FUNCTION_BLOCK FB_Visu
VAR_INPUT
	(***** Sensors to detect boxes *****)
	bBarrierSensor				AT %I*: BOOL;	// True if barrier sensor detects a box
	bMetalSensor				AT %I*: BOOL;	// True if metal sensor detects a metal box
	bPlasticSensor				AT %I*: BOOL;	// True if plastic sensor detects a box
	
	bError						: BOOL;			// True if modules have errors
(***** Axis variables *****)
	lrAxisVelo					: LREAL;
	
(***** State of machine elements *****)
	bComprAirEnabled			: BOOL;			// True if compressed air is enabled
	bPowerEnabled				: BOOL;			// True if power supply is enabled
	bMainAxisMoves				: BOOL;			// True if main axis is moving
	bMetalAxisMoves				: BOOL;			// True if metal axis is moving
	bPlasticAxisMoves			: BOOL;			// True if plastic axis is moving
	bClampToWork				: BOOL;			// True if clamp cylinder moves to work position
	bBarrierToWork				: BOOL;			// True if barrier cylinder moves to work position
	bMetalToWork				: BOOL;			// True if metal cylinder moves to work position
	bPlasticToWork				: BOOL;			// True if plastic cylinder moves to work position
(***** Error *****)
	bClampError					: BOOL;			// True if clamp cylinder has an error
	sClampErrMsg				: STRING;			// Error message of clamp cylinder
	bMetalCylError				: BOOL;			// True if metal cylinder has an error
	sMetalErrMsg				: STRING;			// Error message of metal cylinder
	bPlasticCylError			: BOOL;			// True if plastic cylinder has an error
	sPlasticErrMsg				: STRING;			// Error message of plastic cylinder
	iMainAxisErrorId			: DWORD;			// Error id of main axis
	iMetalAxisErrorId			: DWORD;			// Error id of metal axis
	iPlasticAxisErrorId			: DWORD;			// Error id of plastic axis
	
(***** PS_PackML_StateMachine *****)
	bStarted					: BOOL;			// True if state machine is in state EXECUTE
	bStopped					: BOOL;			// True if state machine is in state STOPPED
	bReset						: BOOL;			// True if state machine is in state RESETTING
	bAborted					: BOOL;			// True if state machine is in state ABORTED
	bIdle						: BOOL;			// True if state machine is in state IDLE
	bAuto						: BOOL;			// True if state machine is in mode AUTOMATIC
	bSemi						: BOOL;			// True if state machine is in mode SEMIAUTOMATIC
	bManual						: BOOL;			// True if state machine is in mode MANUAL
	bMaintenance				: BOOL;			// True if state machine is in mode MAINTENANCE
	bStartButtonOff				: BOOL;			// To turn off start button

(***** Buttons of visualisation - inputs *****)
		(* State buttons *)
	bButtonPowerIn				: BOOL;			// Input signal of power button
	bButtonComprAirIn			: BOOL;			// Input signal of compressed air button
	bButtonStartIn				: BOOL;			// Input signal of start button
	bButtonStopIn				: BOOL;			// Input signal of stop button
	bButtonResetIn				: BOOL;			// Input signal of reset button
	bButtonAbortIn				: BOOL;			// Input signal of abort button
		(* Mode buttons *)
	bButtonAutoIn				: BOOL;			// Input signal of automatic button
	bButtonSemiIn				: BOOL;			// Input signal of semi-automatic button
	bButtonManuIn				: BOOL;			// Input signal of manual button
	bButtonMaintenanceIn		: BOOL;			// Input signal of maintenance button
		(* Axis buttons *)
	bButtonMainFwIn				: BOOL;			// Input signal of button to move main axis forwards
	bButtonMainBwIn				: BOOL;			// Input signal of button to move main axis backwards
	bButtonMetalFwIn			: BOOL;			// Input signal of button to move metal axis forwards
	bButtonMetalBwIn			: BOOL;			// Input signal of button to move metal axis backwards
	bButtonPlasticFwIn			: BOOL;			// Input signal of button to move plastic axis forwards
	bButtonPlasticBwIn			: BOOL;			// Input signal of button to move plastic axis backwards
		(* Cylinder buttons *)
	bButtonClampToWorkIn		: BOOL;			// Input signal of button to move clamp cylinder
	bButtonBarrierToWorkIn		: BOOL;			// Input signal of button to move barrier cylinder
	bButtonMetalToWorkIn		: BOOL;			// Input signal of button to move metal cylinder
	bButtonPlasticToWorkIn		: BOOL;			// Input signal of button to move plastic cylinder
END_VAR
VAR_OUTPUT
	lrYClamp					AT %Q*: LREAL;					// Y-Coordinate of clamp cylinder
	lrYBarrier					AT %Q*: LREAL;					// Y-Coordinate of barrier cylinder
	lrYMetal					AT %Q*: LREAL;					// Y-Coordinate of metal cylinder
	lrYPlastic					AT %Q*: LREAL;					// Y-Coordinate of plastic cylinder
	lrBoxX						AT %Q*: ARRAY[1..4] OF LREAL;	// X-Coordinates of boxes
	lrBoxY						AT %Q*: ARRAY[1..4] OF LREAL;	// Y-Coordinates of boxes
	
(***** Buttons of visualisation - outputs *****)
		(* State buttons *)
	bButtonPowerOut				: BOOL;			// To turn on and off the machine
	bButtonComprAirOut			: BOOL;			// To enable compressed air
	bButtonStartOut				: BOOL;			// To change state into state START
	bButtonStopOut				: BOOL;			// To change state into state STOP
	bButtonResetOut				: BOOL;			// To change state into state RESET
	
		(* Mode buttons *)
	bButtonAutoOut				: BOOL;			// To change mode into mode AUTOMATIC		
	bButtonSemiOut				: BOOL;			// To change mode into mode SEMI-AUTOMATIC	
	bButtonManuOut				: BOOL;			// To change mode into mode MANAUL	
	bButtonMaintenanceOut		: BOOL;			// To change mode into mode MAINTENANCE	
	
		(* Axis buttons *)
	bButtonMainFwOut			: BOOL;			// To move main axis forwards
	bButtonMainBwOut			: BOOL;			// To move main axis backwards
	bButtonMetalFwOut			: BOOL;			// To move metal axis forwards
	bButtonMetalBwOut			: BOOL;			// To move metal axis backwards
	bButtonPlasticFwOut			: BOOL;			// To move plastic axis forwards
	bButtonPlasticBwOut			: BOOL;			// To move plastic axis backwards
	
		(* Cylinder buttons *)
	bButtonClampToWorkOut		: BOOL;			// To move manually clamp cylinder to work position
	bButtonBarrierToWorkOut		: BOOL;			// To move manually barrier cylinder to work position
	bButtonMetalToWorkOut		: BOOL;			// To move manually metal cylinder to work position
	bButtonPlasticToWorkOut		: BOOL;			// To move manually plastic cylinder to work position
END_VAR
VAR
	iBoxesLast					: INT;						// Box on last position of main belt
	bBoxMetalMove				: ARRAY[1..4] OF BOOL;		// bBoxMetalMove[1] is true, if box 1 is moved by metal cylinder
	bBoxMetalFree				: ARRAY[1..4] OF BOOL;		// bBoxMetalFree[1] is true, if any box blockades the metal belt
	bBoxPlasticMove				: ARRAY[1..4] OF BOOL;		// bBoxPlasticMove[1] is true, if box 1 is moved by plastic cylinder
	bBoxPlasticFree				: ARRAY[1..4] OF BOOL;		// bBoxMetalFree[1] is true, if any box blockades the plastic belt
	bBoxMainBelt				: ARRAY[1..4] OF BOOL;		// bBoxMainBelt[1] is true, if box 1 is on main belt and has no
	bBoxMetalBelt				: ARRAY[1..4] OF BOOL;				// obstacles, so box 1 is moved by main axis
	bBoxPlasticBelt				: ARRAY[1..4] OF BOOL;
	lrMainVelo					: LREAL;					// Velocity of boxes on main belt
	lrMetalVelo					: LREAL;					// Velocity of boxes on metal belt
	lrPlasticVelo				: LREAL;					// Velocity of boxes on plastic belt
	bAccident					: BOOL;						// True if machine caused an accident
	iState						: INT;
	
	iMessages					: INT;						// Number of messages
	sMessageClamp				: STRING;					// Message of clamp cylinder
	sMessageMetalCyl			: STRING;					// Message of metal cylinder
	sMessagePlasticCyl			: STRING;					// Message of plastic cylinder
	sMessageMainAxis			: STRING;					// Message of main axis
	sMessageMetalAxis			: STRING;					// Message of metal axis
	sMessagePlasticAxis			: STRING;					// Message of plastic axis
	iAngleMain					: INT;						// Angle of main axis element
	iAngleMetal					: INT;						// Angle of metal axis element
	iAnglePlastic				: INT;						// Angle of plastic axis element
	tonMainAxis					: TON;						// Timer for movement of main axis element
	tonMetalAxis				: TON;						// Timer for movement of metal axis element
	tonPlasticAxis				: TON;						// Timer for movement of plastic axis element

(* ========================== COLOR VARIABLES =============================== *)

	dwYellow					: DWORD;
	dwGreen						: DWORD;
	dwPink						: DWORD;
	dwButtonColorStart			: DWORD;					// Color of start button
	bButtonColorStart			: BOOL;						// To change color of start button
	dwButtonColorStop			: DWORD;					// Color of stop button
	bButtonColorStop			: BOOL;						// To change color of stop button
	dwButtonColorReset			: DWORD;					// Color of reset button
	bButtonColorReset			: BOOL;						// To change color of reset button
	dwButtonColorAuto			: DWORD;					// Color of automatic button
	bButtonColorAuto			: BOOL;						// To change color of automatic button
	dwButtonColorSemi			: DWORD;					// Color of semi-automatic button
	bButtonColorSemi			: BOOL;						// To change color of semi-automatic button
	dwButtonColorManu			: DWORD;					// Color of manual button
	bButtonColorManu			: BOOL;						// To change color of manual button
	dwButtonColorMaint			: DWORD;					// Color of maintenance button
	bButtonColorMaint			: BOOL;						// To change color of maintenance button
	dwButtonColorClamp			: DWORD;					// Color of button to move clamp cylinder
	bButtonColorClamp			: BOOL;						// To change color of clamp button
	dwButtonColorBarrier		: DWORD;					// Color of button to move barrier cylinder
	bButtonColorBarrier			: BOOL;						// To change color of barrier button
	dwButtonColorMetalCyl		: DWORD;					// Color of button to move metal cylinder
	bButtonColorMetalCyl		: BOOL;						// To change color of metal cylinder button
	dwButtonColorPlasticCyl		: DWORD;					// Color of button to move plastic cylinder
	bButtonColorPlasticCyl		: BOOL;						// To change color of plastic cylinder button
	dwButtonColorMainFw			: DWORD;					// Color of button to move main axis forwards
	bButtonColorMainFw			: BOOL;						// To change color of button to move main axis fw.
	dwButtonColorMainBw			: DWORD;					// Color of button to move main axis backwards
	bButtonColorMainBw			: BOOL;						// To change color of button to move main axis bw.
	dwButtonColorMetalFw		: DWORD;					// Color of button to move metal axis forwards
	bButtonColorMetalFw			: BOOL;						// To change color of button to move metal axis fw.
	dwButtonColorMetalBw		: DWORD;					// Color of button to move metal axis backwards
	bButtonColorMetalBw			: BOOL;						// To change color of button to move metal axis bw.
	dwButtonColorPlasticFw		: DWORD;					// Color of button to move plastic axis forwards
	bButtonColorPlasticFw		: BOOL;						// To change color of button to move plastic axis fw.
	dwButtonColorPlasticBw		: DWORD;					// Color of button to move plastic axis backwards
	bButtonColorPlasticBw		: BOOL;						// To change color of button to move plastic axis bw.
	dwButtonColorComprAir		: DWORD;					// Color of button to enable/disable compressed air
	bButtonColorComprAir		: BOOL;						// To change color of button to control compressed air
END_VAR

// =========================================================
	// Resetting visu
	
IF bReset THEN
	M_Reset();
END_IF

// =========================================================
	// Because of the visualisation size
	// the boxes velocity is a fraction of the axis velocity
	
IF bAuto OR bSemi OR bButtonMainFwIn THEN
	lrMainVelo := lrAxisVelo / 250;
ELSIF bButtonMainBwIn THEN
	lrMainVelo := - lrAxisVelo / 250;
END_IF
IF bAuto OR bSemi OR bButtonMetalFwIn THEN
	lrMetalVelo := - lrAxisVelo / 250;
ELSIF bButtonMetalBwIn THEN
	lrMetalVelo := lrAxisVelo / 250;
END_IF
IF bAuto OR bSemi OR bButtonPlasticFwIn THEN
	lrPlasticVelo := - lrAxisVelo / 250;
ELSIF bButtonPlasticBwIn THEN
	lrPlasticVelo := lrAxisVelo / 250;
END_IF

// =========================================================
	// In case of accident the power button is turned off
	
IF bAccident THEN
	IF bButtonPowerOut THEN
		bButtonPowerOut := FALSE;
	END_IF
	IF bStopped THEN
		bAccident := FALSE;
	END_IF
END_IF

// =========================================================
	// Rotation of axis elements
M_AxisRotation();

	// Buttons, order of boxes, error messages
M_ButtonSignals();
M_ButtonColors();
M_LastBox();
M_ErrorMessages();

	// Motion of cylinders
M_Barrier_Clamp_Cyl();
M_Metal_Plastic_Cyl();

	// Motion of boxes
M_AxisMoveBoxes();
M_CylinderMoveBoxes();

// =========================================================

METHOD PRIVATE M_AxisMoveBoxes
VAR_INPUT
END_VAR
// =========================================================
	// Checking traction standby on main belt
	
bBoxMainBelt[1] := lrBoxY[1] >= -5	// box 1 on main belt
						// not previous to box 2											
					AND ((lrBoxX[2] - lrBoxX[1] - lrMainVelo) >= 119.99999 OR (lrBoxX[2] - lrBoxX[1] - lrMainVelo) <= 0.001 OR lrBoxY[2] < -60)
						// not previous to box 3	
					AND ((lrBoxX[3] - lrBoxX[1] - lrMainVelo) >= 179.99999 OR (lrBoxX[3] - lrBoxX[1]- lrMainVelo) <= 60.001 OR lrBoxY[3] < -60)
						// not previous to box 4
					AND ((lrBoxX[4] - lrBoxX[1] - lrMainVelo) >= 239.99999 OR (lrBoxX[4] - lrBoxX[1]- lrMainVelo) <= 120.001 OR lrBoxY[4] < -60);
					
bBoxMainBelt[2] := lrBoxY[2] >= -5
					AND ((lrBoxX[1] - lrBoxX[2] - lrMainVelo) >= -0.00001 OR (lrBoxX[1] - lrBoxX[2] - lrMainVelo) <= -119.999 OR lrBoxY[1] < -60)
					AND ((lrBoxX[3] - lrBoxX[2] - lrMainVelo) >= 119.99999 OR (lrBoxX[3] - lrBoxX[2] - lrMainVelo) <= 0.001 OR lrBoxY[3] < -60)
					AND ((lrBoxX[4] - lrBoxX[2] - lrMainVelo) >= 179.99999 OR (lrBoxX[4] - lrBoxX[2] - lrMainVelo) <= 60.001 OR lrBoxY[4] < -60);

bBoxMainBelt[3] := lrBoxY[3] >= -5
					AND ((lrBoxX[1] - lrBoxX[3] - lrMainVelo) >= -60.00001 OR (lrBoxX[1] - lrBoxX[3] - lrMainVelo) <= -179.999 OR lrBoxY[1] < -60)
					AND ((lrBoxX[2] - lrBoxX[3] - lrMainVelo) >= -0.00001 OR (lrBoxX[2] - lrBoxX[3] - lrMainVelo) <= -119.999 OR lrBoxY[2] < -60)
					AND ((lrBoxX[4] - lrBoxX[3] - lrMainVelo) >= 119.99999 OR (lrBoxX[4] - lrBoxX[3] - lrMainVelo) <= 0.001 OR lrBoxY[4] < -60);
					
bBoxMainBelt[4] := lrBoxY[4] >= -5
					AND ((lrBoxX[1] - lrBoxX[4] - lrMainVelo) >= -120.00001 OR (lrBoxX[1] - lrBoxX[4] - lrMainVelo) <= -239.999 OR lrBoxY[1] < -60)
					AND ((lrBoxX[2] - lrBoxX[4] - lrMainVelo) >= -60.00001 OR (lrBoxX[2] - lrBoxX[4] - lrMainVelo) <= -179.999 OR lrBoxY[2] < -60)
					AND ((lrBoxX[3] - lrBoxX[4] - lrMainVelo) >= -0.00001 OR (lrBoxX[3] - lrBoxX[4] - lrMainVelo) <= -119.999 OR lrBoxY[3] < -60);
					
// =========================================================
	// Motion of boxes on main belt - forwards
					
IF bMainAxisMoves AND (bAuto OR bSemi OR bButtonMainFwIn) THEN
	FOR iState := 1 TO 4 BY 1 DO
		IF bBoxMainBelt[iState] THEN	
				// not previous to moving metal cylinder
			IF lrBoxX[iState] >= (60*iState + 30) AND lrBoxX[iState] < (260 + 60*iState) THEN
				IF lrYMetal <= -9 THEN
					IF lrBoxX[iState] < (131.25 + 60*iState) AND lrBoxX[iState] > (130.95 + 60*iState) THEN
						lrBoxX[iState] := 131 + 60*iState;
					ELSIF lrBoxX[iState] <= (130.95 + 60*iState) THEN
						lrBoxX[iState] := lrBoxX[iState] + lrMainVelo;
					END_IF
				ELSE
					lrBoxX[iState] := lrBoxX[iState] + lrMainVelo;
				END_IF
			END_IF
				// not previous to moving plastic cylinder
			IF lrBoxX[iState] >= (260 + 60*iState) THEN
				IF lrYPlastic <= -9 THEN
					IF lrBoxX[iState] < (381.25 + 60*iState) AND lrBoxX[iState] > (380.95 + 60*iState) THEN
						lrBoxX[iState] := 381 + 60*iState;
					ELSIF lrBoxX[iState] <= (380.95 + 60*iState) THEN
						lrBoxX[iState] := lrBoxX[iState] + lrMainVelo;
					END_IF
				ELSE
					lrBoxX[iState] := lrBoxX[iState] + lrMainVelo;
				END_IF
			END_IF
				// barrier open and box 1 in the first place
			IF lrYBarrier >= 61 AND lrBoxX[iState] >= 60*(iState - 1) AND lrBoxX[iState] <  (60*iState + 30) THEN
				IF lrBoxX[iState] + lrMainVelo < (60*iState + 30) THEN
					 lrBoxX[iState] := lrBoxX[iState] + lrMainVelo;
				ELSIF lrBoxX[iState] < (60*iState + 30) THEN
					lrBoxX[iState] := (60*iState + 30);
				END_IF
			END_IF	
				// not previous to clamp
			IF lrBoxX[iState] + lrMainVelo < -60*(3 - iState) THEN
				lrBoxX[iState] := lrBoxX[iState] + lrMainVelo;
			ELSIF lrBoxX[iState] < -60*(iState + 1) THEN
				lrBoxX[iState] := -60*(iState + 1);
			END_IF
				// clamp open, not after clamp											
			IF lrYClamp >= 1 AND lrBoxX[iState] >= -60*(iState + 1) THEN
				IF lrBoxX[iState] + lrMainVelo < 60*(iState - 1) THEN
					lrBoxX[iState] := lrBoxX[iState] + lrMainVelo;
				ELSIF lrBoxX[iState] < 60*(iState - 1) THEN
					lrBoxX[iState] := 60*(iState - 1);
				END_IF
			END_IF
		END_IF
	END_FOR
END_IF

// =========================================================
	// Motion of boxes on main belt - backwards
	
IF bMainAxisMoves AND bButtonMainBwIn THEN 
	FOR iState := 1 TO 4 BY 1 DO
		IF bBoxMainBelt[iState] THEN
				// not previous to moving metal cylinder
			IF lrBoxX[iState] >= (90 + 60*iState) AND lrBoxX[iState] < (262 + 60*iState) THEN
				IF NOT (lrBoxX[iState] < (261.25 + 60*iState) AND lrBoxX[iState] > (260.95 + 60*iState) AND lrYMetal <= -9) THEN
					lrBoxX[iState] := lrBoxX[iState] + lrMainVelo;
				ELSE
					lrBoxX[iState] := 261 + 60*iState;
				END_IF
			END_IF
				// not previous to moving plastic cylinder
			IF lrBoxX[iState] >=  (262 + 60*iState) THEN
				lrBoxX[iState] := lrBoxX[iState] + lrMainVelo;
			END_IF
				// not previous to moving barrier cylinder
			IF lrBoxX[iState] > 60*(iState - 1) AND lrBoxX[iState] < (90 + 60*iState) THEN
				IF NOT (lrBoxX[iState] < (30.25 + 60*iState) AND lrBoxX[iState] > (29.95 + 60*iState) AND lrYBarrier < 61) THEN
					lrBoxX[iState] := lrBoxX[iState] + lrMainVelo;
				ELSE
					lrBoxX[iState] := 60*iState + 30;
				END_IF
			END_IF
				// barrier open and box 1 after the first place
			IF lrYBarrier >= 61 AND lrBoxX[iState] < 60*(iState + 1) AND lrBoxX[iState] > 60*(iState - 1) THEN
				lrBoxX[iState] := lrBoxX[iState] + lrMainVelo;
			END_IF	
				// clamp open, not previous to clamp											
			IF lrYClamp >= 1 AND lrBoxX[iState] <= 60*(iState-1) AND lrBoxX[iState] > -60*(3-iState) THEN
				lrBoxX[iState] := lrBoxX[iState] + lrMainVelo;
			END_IF
				// not at the beginning of main belt
			IF lrBoxX[iState] > -60*(4-iState) AND lrBoxX[iState] <= -60*(3-iState) THEN
				lrBoxX[iState] := lrBoxX[iState] + lrMainVelo;
			END_IF
		END_IF
	END_FOR	
END_IF

// =========================================================
// =========================================================
	// Checking traction standby on metal belt
	
bBoxMetalBelt[1] := lrBoxX[1] > 240 AND lrBoxX[1] <= 271	// box 1 on metal belt
						// not previous to box 2											
					AND ((lrBoxY[2] - lrBoxY[1] - lrMetalVelo) >= 60 OR (lrBoxY[2] - lrBoxY[1] - lrMetalVelo) <= -60
							OR NOT (lrBoxX[2] > 300 AND lrBoxX[2] <= 331))
						// not previous to box 3	
					AND ((lrBoxY[3] - lrBoxY[1]- lrMetalVelo) >= 60 OR (lrBoxY[3] - lrBoxY[1]- lrMetalVelo) <= -60
							OR NOT (lrBoxX[3] > 360 AND lrBoxX[3] <= 391))
						// not previous to box 4
					AND ((lrBoxY[4] - lrBoxY[1]- lrMetalVelo) >= 60 OR (lrBoxY[4] - lrBoxY[1]- lrMetalVelo) <= -60
							OR NOT (lrBoxX[4] > 420 AND lrBoxX[4] <= 451));	
					
bBoxMetalBelt[2] := lrBoxX[2] > 300 AND lrBoxX[2] <= 331										
					AND ((lrBoxY[1] - lrBoxY[2] - lrMetalVelo) >= 60 OR (lrBoxY[1] - lrBoxY[2] - lrMetalVelo) <= -60
							OR NOT (lrBoxX[1] > 240 AND lrBoxX[1] <= 271))
					AND ((lrBoxY[3] - lrBoxY[2]- lrMetalVelo) >= 60 OR (lrBoxY[3] - lrBoxY[2]- lrMetalVelo) <= -60
							OR NOT (lrBoxX[3] > 360 AND lrBoxX[3] <= 391))
					AND ((lrBoxY[4] - lrBoxY[2]- lrMetalVelo) >= 60 OR (lrBoxY[4] - lrBoxY[2]- lrMetalVelo) <= -60
							OR NOT (lrBoxX[4] > 420 AND lrBoxX[4] <= 451));	
					
bBoxMetalBelt[3] := lrBoxX[3] > 360 AND lrBoxX[3] <= 391										
					AND ((lrBoxY[1] - lrBoxY[3] - lrMetalVelo) >= 60 OR (lrBoxY[1] - lrBoxY[3] - lrMetalVelo) <= -60
							OR NOT (lrBoxX[1] > 240 AND lrBoxX[1] <= 271))
					AND ((lrBoxY[2] - lrBoxY[3]- lrMetalVelo) >= 60 OR (lrBoxY[2] - lrBoxY[3]- lrMetalVelo) <= -60
							OR NOT (lrBoxX[2] > 300 AND lrBoxX[2] <= 331))
					AND ((lrBoxY[4] - lrBoxY[3]- lrMetalVelo) >= 60 OR (lrBoxY[4] - lrBoxY[3]- lrMetalVelo) <= -60
							OR NOT (lrBoxX[4] > 420 AND lrBoxX[4] <= 451));	
					
bBoxMetalBelt[4] := lrBoxX[4] > 420 AND lrBoxX[4] <= 451										
					AND ((lrBoxY[1] - lrBoxY[4] - lrMetalVelo) >= 60 OR (lrBoxY[1] - lrBoxY[4] - lrMetalVelo) <= -60
							OR NOT (lrBoxX[1] > 240 AND lrBoxX[1] <= 271))
					AND ((lrBoxY[2] - lrBoxY[4] - lrMetalVelo) >= 60 OR (lrBoxY[2] - lrBoxY[4] - lrMetalVelo) <= -60
							OR NOT (lrBoxX[2] > 300 AND lrBoxX[2] <= 331))
					AND ((lrBoxY[3] - lrBoxY[4]- lrMetalVelo) >= 60 OR (lrBoxY[3] - lrBoxY[4]- lrMetalVelo) <= -60
							OR NOT (lrBoxX[3] > 360 AND lrBoxX[3] <= 391));

// =========================================================
	// Motion of boxes on metal belt and back to the start position number 4
	
FOR iState := 1 TO 4 BY 1 DO	
	IF bMetalAxisMoves THEN
		IF 	bBoxMetalBelt[iState] THEN
		(* Check the state and direction of motion *)		
				IF bAuto OR bSemi OR (NOT bAuto AND bButtonMetalFwIn) THEN
				(* Move box to the end of metal belt and then back to position 4 *)	
					IF lrBoxY[iState] <= -64.9 AND lrBoxY[iState] > -140.0 THEN
						lrBoxY[iState] := lrBoxY[iState] + lrMetalVelo;
					END_IF
				ELSIF NOT bAuto AND bButtonMetalBwIn THEN
					IF lrBoxY[iState] + lrMetalVelo <= -65.1 THEN
						lrBoxY[iState] := lrBoxY[iState] + lrMetalVelo;
					END_IF
				END_IF
		END_IF
	END_IF	
	
	IF lrBoxY[iState] <= -140.0 AND iBoxesLast = 0 THEN
		lrBoxY[iState] := 0;
		lrBoxX[iState] := -240 + iState*60;
	END_IF
END_FOR
	
// =========================================================
// =========================================================
	// Checking traction standby on plastic belt
	
bBoxPlasticBelt[1] := lrBoxX[1] > 470 AND lrBoxX[1] <= 521	// box 1 on plastic belt
						// not previous to box 2											
					AND ((lrBoxY[2] - lrBoxY[1] - lrPlasticVelo) >= 60 OR (lrBoxY[2] - lrBoxY[1] - lrPlasticVelo) <= -60
							OR NOT (lrBoxX[2] > 530 AND lrBoxX[2] <= 581))
						// not previous to box 3	
					AND ((lrBoxY[3] - lrBoxY[1]- lrPlasticVelo) >= 60 OR (lrBoxY[3] - lrBoxY[1]- lrPlasticVelo) <= -60
							OR NOT (lrBoxX[3] > 590 AND lrBoxX[3] <= 641))
						// not previous to box 4
					AND ((lrBoxY[4] - lrBoxY[1]- lrPlasticVelo) >= 60 OR (lrBoxY[4] - lrBoxY[1]- lrPlasticVelo) <= -60
							OR NOT (lrBoxX[4] > 650 AND lrBoxX[4] <= 701));	
					
bBoxPlasticBelt[2] := lrBoxX[2] > 530 AND lrBoxX[2] <= 581										
					AND ((lrBoxY[1] - lrBoxY[2] - lrPlasticVelo) >= 60 OR (lrBoxY[1] - lrBoxY[2] - lrPlasticVelo) <= -60
							OR NOT (lrBoxX[1] > 470 AND lrBoxX[1] <= 521))
					AND ((lrBoxY[3] - lrBoxY[2]- lrPlasticVelo) >= 60 OR (lrBoxY[3] - lrBoxY[2]- lrPlasticVelo) <= -60
							OR NOT (lrBoxX[3] > 590 AND lrBoxX[3] <= 641))
					AND ((lrBoxY[4] - lrBoxY[2]- lrPlasticVelo) >= 60 OR (lrBoxY[4] - lrBoxY[2]- lrPlasticVelo) <= -60
							OR NOT (lrBoxX[4] > 650 AND lrBoxX[4] <= 701));	
					
bBoxPlasticBelt[3] := lrBoxX[3] > 590 AND lrBoxX[3] <= 641										
					AND ((lrBoxY[1] - lrBoxY[3] - lrPlasticVelo) >= 60 OR (lrBoxY[1] - lrBoxY[3] - lrPlasticVelo) <= -60
							OR NOT (lrBoxX[1] > 470 AND lrBoxX[1] <= 521))
					AND ((lrBoxY[2] - lrBoxY[3]- lrPlasticVelo) >= 60 OR (lrBoxY[2] - lrBoxY[3]- lrPlasticVelo) <= -60
							OR NOT (lrBoxX[2] > 530 AND lrBoxX[2] <= 581))
					AND ((lrBoxY[4] - lrBoxY[3]- lrPlasticVelo) >= 60 OR (lrBoxY[4] - lrBoxY[3]- lrPlasticVelo) <= -60
							OR NOT (lrBoxX[4] > 650 AND lrBoxX[4] <= 701));	
					
bBoxPlasticBelt[4] := lrBoxX[4] > 650 AND lrBoxX[4] <= 701										
					AND ((lrBoxY[1] - lrBoxY[4] - lrPlasticVelo) >= 60 OR (lrBoxY[1] - lrBoxY[4] - lrPlasticVelo) <= -60
							OR NOT (lrBoxX[1] > 470 AND lrBoxX[1] <= 521))
					AND ((lrBoxY[2] - lrBoxY[4] - lrPlasticVelo) >= 60 OR (lrBoxY[2] - lrBoxY[4] - lrPlasticVelo) <= -60
							OR NOT (lrBoxX[2] > 530 AND lrBoxX[2] <= 581))
					AND ((lrBoxY[3] - lrBoxY[4]- lrPlasticVelo) >= 60 OR (lrBoxY[3] - lrBoxY[4]- lrPlasticVelo) <= -60
							OR NOT (lrBoxX[3] > 590 AND lrBoxX[3] <= 641));

// =========================================================
	// Motion of boxes on metal belt and back to the start position number 4

FOR iState := 1 TO 4 BY 1 DO	
	IF bPlasticAxisMoves THEN
			IF 	bBoxPlasticBelt[iState] THEN	
				(* Check the state and direction of motion *)		
				IF bAuto OR bSemi OR (NOT bAuto AND bButtonPlasticFwIn) THEN
				(* Move box to the end of metal belt and then back to position 4 *)	
					IF lrBoxY[iState] <= -64.9 AND lrBoxY[iState] > -140.0 THEN
							lrBoxY[iState] := lrBoxY[iState] + lrPlasticVelo;
					END_IF
				ELSIF NOT bAuto AND bButtonPlasticBwIn THEN
					IF lrBoxY[iState] + lrPlasticVelo <= -65.1 THEN
						lrBoxY[iState] := lrBoxY[iState] + lrPlasticVelo;
					END_IF
				END_IF
			END_IF
	END_IF
	
	IF lrBoxY[iState] <= -140.0 AND iBoxesLast = 0 THEN
		lrBoxY[iState] := 0;
		lrBoxX[iState] := -240 + iState*60;
	END_IF
END_FOR

// =========================================================
END_METHOD

METHOD PRIVATE M_AxisRotation
VAR_INPUT
END_VAR
// =========================================================
	// Rotation of main axis
	
tonMainAxis( IN := bMainAxisMoves,
			 PT := T#0.04S );

IF tonMainAxis.Q THEN
	tonMainAxis( IN := FALSE );
	IF bAuto OR bSemi THEN
		iAngleMain := iAngleMain + 2;
	ELSIF bButtonMainFwIn THEN
		iAngleMain := iAngleMain + 1;
	ELSIF bButtonMainBwIn THEN
		iAngleMain := iAngleMain - 1;
	END_IF
END_IF

// =========================================================
	// Rotation of metal axis
	
tonMetalAxis( IN := bMetalAxisMoves,
			 PT := T#0.04S );

IF tonMetalAxis.Q THEN
	tonMetalAxis( IN := FALSE );
	IF bAuto OR bSemi THEN
		iAngleMetal := iAngleMetal + 2;
	ELSIF bButtonMetalFwIn THEN
		iAngleMetal := iAngleMetal + 1;
	ELSIF bButtonMetalBwIn THEN
		iAngleMetal := iAngleMetal - 1;
	END_IF
END_IF

// =========================================================
	// Rotation of plastic axis
	
tonPlasticAxis( IN := bPlasticAxisMoves,
			 PT := T#0.04S );

IF tonPlasticAxis.Q THEN
	tonPlasticAxis( IN := FALSE );
	IF bAuto OR bSemi THEN
		iAnglePlastic := iAnglePlastic + 2;
	ELSIF bButtonPlasticFwIn THEN
		iAnglePlastic := iAnglePlastic + 1;
	ELSIF bButtonPlasticBwIn THEN
		iAnglePlastic := iAnglePlastic - 1;
	END_IF
END_IF

// =========================================================
END_METHOD

METHOD PRIVATE M_Barrier_Clamp_Cyl
VAR_INPUT
END_VAR
// =========================================================
	// Moving clamp cylinder
	
IF bClampToWork THEN
	IF (lrYClamp + 0.1) < 3.0 THEN
		lrYClamp := lrYClamp + 0.1;
	ELSE
		lrYClamp := 3.0;
	END_IF
ELSE
	IF (lrYClamp - 0.1) > 0.0 THEN
		lrYClamp := lrYClamp - 0.1;
	ELSE
		lrYClamp := 0.0;
	END_IF
END_IF

// =========================================================
// =========================================================
	// Moving barrier cylinder
	
IF bBarrierToWork THEN
	IF (lrYBarrier + 1) < 63.0 THEN
		lrYBarrier := lrYBarrier + 1;
	ELSE
		lrYBarrier := 63.0;
	END_IF
ELSE
	IF (lrYBarrier - 1) > 0.0 THEN
		lrYBarrier := lrYBarrier - 1;
	ELSE
		lrYBarrier := 0.0;
	END_IF
END_IF

// =========================================================
	// Checking position of boxes related to the barrier cylinder
	
IF lrYBarrier <= 60 AND NOT bBarrierToWork THEN
	FOR iState := 1 TO 4 BY 1 DO
		IF lrBoxX[iState] > (-59.89 + 60*iState) AND lrBoxX[iState] < (60*iState + 30) AND lrBoxY[iState] = 0
			AND NOT bStopped THEN
				bAccident := TRUE;
		END_IF
	END_FOR
END_IF

// =========================================================
END_METHOD

METHOD PRIVATE M_ButtonColors
VAR_INPUT
END_VAR
// =========================================================
		// Colors
		
dwYellow := 16#00FFFF80;
dwGreen := 16#0080FF00;
dwPink := 16#00FF8080;

// =========================================================
		// Start button
		
IF (bAccident OR (bPowerEnabled AND (NOT bStarted OR (bSemi AND bStarted))
	AND NOT bButtonStopIn AND NOT bButtonAbortIn AND NOT bButtonResetIn
	AND (bAuto OR bSemi OR bManual OR bMaintenance))) AND NOT (bError AND bIdle) THEN
		IF bButtonStartOut THEN
			dwButtonColorStart := dwGreen;
		ELSE
			dwButtonColorStart := dwYellow;
		END_IF
		bButtonColorStart := TRUE;
ELSE
	bButtonColorStart := FALSE;
END_IF

// =========================================================
		// Stop button
		
IF (bStarted OR bIdle) AND (bAuto OR bSemi OR bManual OR bMaintenance) THEN
	IF bButtonStopOut THEN
		dwButtonColorStop := dwGreen;
	ELSE
		dwButtonColorStop := dwYellow;
	END_IF
	bButtonColorStop := TRUE;
ELSE
	bButtonColorStop := FALSE;
END_IF

// =========================================================
		// Reset button
		
IF bStopped AND bPowerEnabled THEN
	IF bButtonResetOut THEN
		dwButtonColorReset := dwGreen;
	ELSE
		dwButtonColorReset := dwYellow;		
	END_IF
	bButtonColorReset := TRUE;
ELSE
	bButtonColorReset := FALSE;
END_IF

// =========================================================
		// Mode buttons

IF bPowerEnabled THEN
	IF NOT bAuto THEN
		IF bIdle THEN
			dwButtonColorAuto := dwYellow;
			bButtonColorAuto := TRUE;
		ELSE
			bButtonColorAuto := FALSE;
		END_IF
	ELSE
		dwButtonColorAuto := dwGreen;
		bButtonColorAuto := TRUE;
	END_IF
	
	IF NOT bSemi THEN
		IF bIdle THEN
			dwButtonColorSemi := dwYellow;
			bButtonColorSemi := TRUE;
		ELSE
			bButtonColorSemi := FALSE;
		END_IF
	ELSE
		dwButtonColorSemi := dwGreen;
		bButtonColorSemi := TRUE;
	END_IF
	
	IF NOT bManual THEN
		IF bIdle THEN
			dwButtonColorManu := dwYellow;
			bButtonColorManu := TRUE;
		ELSE
			bButtonColorManu := FALSE;
		END_IF
	ELSE
		dwButtonColorManu := dwGreen;
		bButtonColorManu := TRUE;
	END_IF
	
	IF NOT bMaintenance THEN
		IF bIdle THEN
			dwButtonColorMaint := dwYellow;
			bButtonColorMaint := TRUE;
		ELSE
			bButtonColorMaint := FALSE;
		END_IF
	ELSE
		dwButtonColorMaint := dwGreen;
		bButtonColorMaint := TRUE;
	END_IF
END_IF

// =========================================================
		// Buttons to move cylinders and axes
		
IF (bManual OR bMaintenance) AND bStarted THEN
// Cylinders
	IF bButtonClampToWorkOut THEN
		dwButtonColorClamp := dwPink;
	ELSE
		dwButtonColorClamp := dwYellow;
	END_IF
	IF bButtonBarrierToWorkOut THEN
		dwButtonColorBarrier := dwPink;
	ELSE
		dwButtonColorBarrier := dwYellow;
	END_IF
	IF bButtonMetalToWorkOut THEN
		dwButtonColorMetalCyl := dwPink;
	ELSE
		dwButtonColorMetalCyl := dwYellow;
	END_IF
	IF bButtonPlasticToWorkOut THEN
		dwButtonColorPlasticCyl := dwPink;
	ELSE
		dwButtonColorPlasticCyl := dwYellow;
	END_IF
	bButtonColorClamp := TRUE;
	bButtonColorBarrier := TRUE;
	bButtonColorMetalCyl := TRUE;
	bButtonColorPlasticCyl := TRUE;
	
// Axes
	IF bButtonMainBwOut THEN
		dwButtonColorMainBw := dwPink;
	ELSE
		dwButtonColorMainBw := dwYellow;
	END_IF
	IF bButtonMainFwOut THEN
		dwButtonColorMainFw := dwPink;
	ELSE
		dwButtonColorMainFw := dwYellow;
	END_IF
	
	IF bButtonMetalBwOut THEN
		dwButtonColorMetalBw := dwPink;
	ELSE
		dwButtonColorMetalBw := dwYellow;
	END_IF
	IF bButtonMetalFwOut THEN
		dwButtonColorMetalFw := dwPink;
	ELSE
		dwButtonColorMetalFw := dwYellow;
	END_IF
	
	IF bButtonPlasticBwOut THEN
		dwButtonColorPlasticBw := dwPink;
	ELSE
		dwButtonColorPlasticBw := dwYellow;
	END_IF
	IF bButtonPlasticFwOut THEN
		dwButtonColorPlasticFw := dwPink;
	ELSE
		dwButtonColorPlasticFw := dwYellow;
	END_IF
	
	bButtonColorMainBw := NOT bButtonMainFwOut;
	bButtonColorMainFw := NOT bButtonMainBwOut;
	bButtonColorMetalBw := NOT bButtonMetalFwOut;
	bButtonColorMetalFw := NOT bButtonMetalBwOut;
	bButtonColorPlasticBw := NOT bButtonPlasticFwOut;
	bButtonColorPlasticFw := NOT bButtonPlasticBwOut;
ELSE
	bButtonColorClamp := FALSE;
	bButtonColorBarrier := FALSE;
	bButtonColorMetalCyl := FALSE;
	bButtonColorPlasticCyl := FALSE;
	bButtonColorMainBw := FALSE;
	bButtonColorMainFw := FALSE;
	bButtonColorMetalBw := FALSE;
	bButtonColorMetalFw := FALSE;
	bButtonColorPlasticBw := FALSE;
	bButtonColorPlasticFw := FALSE;
END_IF
		
// =========================================================
		// Button to control compressed air
		
IF bMaintenance AND bStarted THEN
	IF bButtonComprAirIn THEN
		dwButtonColorComprAir := dwGreen;
	ELSE
		dwButtonColorComprAir := dwYellow;
	END_IF
	bButtonColorComprAir := TRUE;
ELSE
	bButtonColorComprAir := FALSE;
END_IF

// =========================================================
END_METHOD

METHOD PRIVATE M_ButtonSignals
VAR_INPUT
END_VAR
// =========================================================
	// When machine is in requested state, buttons are turned off again

IF bStartButtonOff THEN
	bButtonStartOut := FALSE;
END_IF

IF bStopped THEN
	bButtonStopOut := FALSE;
END_IF

IF bReset THEN
	bButtonResetOut := FALSE;
END_IF

IF bManual THEN
	bButtonManuOut := FALSE;
END_IF

IF bAuto THEN
	bButtonAutoOut := FALSE;
END_IF

IF bSemi THEN
	bButtonSemiOut := FALSE;
END_IF

IF bMaintenance THEN
	bButtonMaintenanceOut := FALSE;
END_IF

// =========================================================
END_METHOD

METHOD PRIVATE M_CylinderMoveBoxes
VAR_INPUT
END_VAR
// =========================================================
	// Metal cylinder - checking the positions of boxes
	
bBoxMetalFree[1] := NOT (lrBoxX[2] > 300 AND lrBoxX[2] <= 331 AND lrBoxY[1] - lrBoxY[2] <= 61)
					AND NOT (lrBoxX[3] > 360 AND lrBoxX[3] <= 391 AND lrBoxY[1] - lrBoxY[3] <= 61)
					AND NOT (lrBoxX[4] > 420 AND lrBoxX[4] <= 451 AND lrBoxY[1] - lrBoxY[4] <= 61);

bBoxMetalFree[2] := NOT (lrBoxX[1] > 240 AND lrBoxX[1] <= 271 AND lrBoxY[2] - lrBoxY[1] <= 61)
					AND NOT (lrBoxX[3] > 360 AND lrBoxX[3] <= 391 AND lrBoxY[2] - lrBoxY[3] <= 61)
					AND NOT (lrBoxX[4] > 420 AND lrBoxX[4] <= 451 AND lrBoxY[2] - lrBoxY[4] <= 61);
					
bBoxMetalFree[3] := NOT (lrBoxX[1] > 240 AND lrBoxX[1] <= 271 AND lrBoxY[3] - lrBoxY[1] <= 61)
					AND NOT (lrBoxX[2] > 300 AND lrBoxX[2] <= 331 AND lrBoxY[3] - lrBoxY[2] <= 61)
					AND NOT (lrBoxX[4] > 420 AND lrBoxX[4] <= 451 AND lrBoxY[3] - lrBoxY[4] <= 61);
					
bBoxMetalFree[4] := NOT (lrBoxX[1] > 240 AND lrBoxX[1] <= 271 AND lrBoxY[4] - lrBoxY[1] <= 61)
					AND NOT (lrBoxX[2] > 300 AND lrBoxX[2] <= 331 AND lrBoxY[4] - lrBoxY[2] <= 61)
					AND NOT (lrBoxX[3] > 360 AND lrBoxX[3] <= 391 AND lrBoxY[4] - lrBoxY[3] <= 61);

// =========================================================
	// Metal cylinder - boxes motion
	
FOR iState := 1 TO 4 BY 1 DO
	IF bMetalToWork AND bBoxMetalMove[iState] AND bBoxMetalFree[iState] THEN
		IF (lrYMetal - 1) >= -72 THEN
			lrYMetal := lrYMetal - 1;
			IF lrYMetal - lrBoxY[iState] <= -9 THEN
				lrBoxY[iState] := lrBoxY[iState] - 1;
			END_IF
		ELSIF lrYMetal = -72 AND (lrYMetal - lrBoxY[iState]) <= -9 THEN
			lrBoxY[iState] := lrBoxY[iState] - 2;
		ELSE
			bBoxMetalMove[iState] := FALSE;
		END_IF
	END_IF	
END_FOR

// =========================================================
// =========================================================
	// Plastic cylinder - checking the positions of boxes

bBoxPlasticFree[1] := NOT (lrBoxX[2] > 550 AND lrBoxX[2] <= 581 AND lrBoxY[1] - lrBoxY[2] <= 61)
					AND NOT (lrBoxX[3] > 610 AND lrBoxX[3] <= 641 AND lrBoxY[1] - lrBoxY[3] <= 61)
					AND NOT (lrBoxX[4] > 670 AND lrBoxX[4] <= 701 AND lrBoxY[1] - lrBoxY[4] <= 61);

bBoxPlasticFree[2] := NOT (lrBoxX[1] > 490 AND lrBoxX[1] <= 521 AND lrBoxY[2] - lrBoxY[1] <= 61)
					AND NOT (lrBoxX[3] > 610 AND lrBoxX[3] <= 641 AND lrBoxY[2] - lrBoxY[3] <= 61)
					AND NOT (lrBoxX[4] > 670 AND lrBoxX[4] <= 701 AND lrBoxY[2] - lrBoxY[4] <= 61);
					
bBoxPlasticFree[3] := NOT (lrBoxX[1] > 490 AND lrBoxX[1] <= 521 AND lrBoxY[3] - lrBoxY[1] <= 61)
					AND NOT (lrBoxX[2] > 550 AND lrBoxX[2] <= 581 AND lrBoxY[3] - lrBoxY[2] <= 61)
					AND NOT (lrBoxX[4] > 670 AND lrBoxX[4] <= 701 AND lrBoxY[3] - lrBoxY[4] <= 61);
					
bBoxPlasticFree[4] := NOT (lrBoxX[1] > 490 AND lrBoxX[1] <= 521 AND lrBoxY[4] - lrBoxY[1] <= 61)
					AND NOT (lrBoxX[2] > 550 AND lrBoxX[2] <= 581 AND lrBoxY[4] - lrBoxY[2] <= 61)
					AND NOT (lrBoxX[3] > 610 AND lrBoxX[3] <= 641 AND lrBoxY[4] - lrBoxY[3] <= 61);
					
// =========================================================
	// Plastic cylinder - boxes motion

FOR iState := 1 TO 4 BY 1 DO
	IF bPlasticToWork AND bBoxPlasticMove[iState] AND bBoxPlasticFree[iState] THEN
		IF (lrYPlastic - 1) >= -72 THEN
			lrYPlastic := lrYPlastic - 1;
			IF lrYPlastic - lrBoxY[iState] <= -9 THEN
				lrBoxY[iState] := lrBoxY[iState] - 1;
			END_IF
		ELSIF lrYPlastic = -72 AND (lrYPlastic - lrBoxY[iState]) <= -9 THEN
			lrBoxY[iState] := lrBoxY[iState] - 2;
		ELSE
			bBoxPlasticMove[iState] := FALSE;
		END_IF
	END_IF	
END_FOR

// =========================================================
END_METHOD

METHOD PRIVATE M_ErrorMessages
VAR_INPUT
END_VAR
// =========================================================
	// Error messages
	
iMessages := 0;
	
IF iMainAxisErrorId = 0 THEN
	sMessageMainAxis := '';
ELSE
	iMessages := iMessages + 1;
	sMessageMainAxis := CONCAT('Error ID of main axis: ', DWORD_TO_STRING(iMainAxisErrorId));
END_IF
// =========================================================
IF iMetalAxisErrorId = 0 THEN
	sMessageMetalAxis := '';
ELSE
	iMessages := iMessages + 1;
	sMessageMetalAxis := CONCAT('Error ID of metal axis: ', DWORD_TO_STRING(iMetalAxisErrorId));
END_IF
// =========================================================
IF iPlasticAxisErrorId = 0 THEN
	sMessagePlasticAxis := '';
ELSE
	iMessages := iMessages + 1;
	sMessagePlasticAxis := CONCAT('Error ID of plastic axis: ', DWORD_TO_STRING(iPlasticAxisErrorId));
END_IF
// =========================================================
IF bClampError THEN
	iMessages := iMessages + 1;
	sMessageClamp := CONCAT('Error of clamp cylinder: ', sClampErrMsg);
ELSE
	sMessageClamp := '';
END_IF
// =========================================================
IF bMetalCylError THEN
	iMessages := iMessages + 1;
	sMessageMetalCyl := CONCAT('Error of metal cylinder: ', sMetalErrMsg);
ELSE
	sMessageMetalCyl := '';
END_IF
// =========================================================
IF bPlasticCylError THEN
	iMessages := iMessages + 1;
	sMessagePlasticCyl := CONCAT('Error of plastic cylinder: ', sPlasticErrMsg);
ELSE
	sMessagePlasticCyl := '';
END_IF
// =========================================================
END_METHOD

METHOD PRIVATE M_LastBox
VAR_INPUT
END_VAR
// =========================================================
	// Checking the last position on main belt

IF lrBoxX[1] >= -180.05 AND lrBoxX[1] < -120.05 AND lrBoxY[1] = 0 THEN
	iBoxesLast := 1;
ELSIF lrBoxX[2] >= -120.05 AND lrBoxX[2] < -60.1 AND lrBoxY[2] = 0 THEN
	iBoxesLast := 2;	
ELSIF lrBoxX[3] >= -60.05 AND lrBoxX[3] < -0.05 AND lrBoxY[3] = 0 THEN
	iBoxesLast := 3;	
ELSIF lrBoxX[4] >= -0.05 AND lrBoxX[4] < 59.95 AND lrBoxY[4] = 0 THEN
	iBoxesLast := 4;	
ELSE
	iBoxesLast := 0;
END_IF		

// =========================================================
END_METHOD

METHOD PRIVATE M_Metal_Plastic_Cyl
VAR_INPUT
END_VAR
// =========================================================
	// Moving metal cylinder
	
IF bMetalToWork THEN
	IF NOT (bBoxMetalMove[1] OR bBoxMetalMove[2] OR bBoxMetalMove[3] OR bBoxMetalMove[4]) THEN
		IF (lrYMetal - 1) >= -73 THEN
			lrYMetal := lrYMetal - 1;
		END_IF
	ELSE
		FOR iState := 1 TO 4 BY 1 DO
			IF bBoxMetalMove[iState] THEN
				IF (lrYMetal - 1) >= (lrBoxY[iState] - 9.1) AND (lrYMetal - 1) >= -73 THEN
					lrYMetal := lrYMetal - 1;
				END_IF
			END_IF
		END_FOR
	END_IF
ELSE
	IF (lrYMetal + 1) < 0.0 THEN
		lrYMetal := lrYMetal + 1;
	ELSE
		lrYMetal := 0.0;
	END_IF
END_IF

// =========================================================
	// Checking position of boxes related to the metal cylinder
	
IF lrYMetal < -8.9 AND lrYMetal > -9.1 AND bMetalToWork THEN
	FOR iState := 1 TO 4 BY 1 DO
			// box on main belt
		IF lrBoxY[iState] >= -5 THEN
				// box in right position related to the metal cylinder
			IF lrBoxX[iState] > (180 + 60*iState) AND lrBoxX[iState] <= (211 + 60*iState) THEN
					bBoxMetalMove[iState] := TRUE;
			END_IF
				// box in wrong position related to the metal cylinder >> accident
			IF ((lrBoxX[iState] > (131 + 60*iState) AND lrBoxX[iState] <= (180 + 60*iState))
				OR (lrBoxX[iState] > (211 + 60*iState) AND lrBoxX[iState] < (261 + 60*iState)))
				AND NOT bStopped THEN
					bAccident := TRUE;
			END_IF
		END_IF
	END_FOR
END_IF

// =========================================================
// =========================================================
	// Moving plastic cylinder
	
IF bPlasticToWork THEN
	IF NOT (bBoxPlasticMove[1] OR bBoxPlasticMove[2] OR bBoxPlasticMove[3] OR bBoxPlasticMove[4]) THEN
		IF (lrYPlastic - 1) >= -73 THEN
			lrYPlastic := lrYPlastic - 1;
		END_IF
	ELSE
		FOR iState := 1 TO 4 BY 1 DO
			IF bBoxPlasticMove[iState] THEN
				IF (lrYPlastic - 1) >= (lrBoxY[iState] - 9.1) AND (lrYPlastic - 1) >= -73 THEN
					lrYPlastic := lrYPlastic - 1;
				END_IF
			END_IF
		END_FOR
	END_IF
ELSE
	IF (lrYPlastic + 1) < 0 THEN
		lrYPlastic := lrYPlastic + 1;
	ELSE
		lrYPlastic := 0;
	END_IF
END_IF

// =========================================================
	// Checking position of boxes related to the plastic cylinder
	
IF (lrBoxX[1] > 521 OR lrBoxX[2] > 581 OR lrBoxX[3] > 641 OR lrBoxX[4] > 701)
	AND NOT bStopped THEN
		bAccident := TRUE;
END_IF
	
IF lrYPlastic < -8.9 AND lrYPlastic > -9.1 AND bPlasticToWork THEN
	FOR iState := 1 TO 4 BY 1 DO
			// box on main belt
		IF lrBoxY[iState] >= -5 THEN
				// box in right position related to the plastic cylinder
			IF lrBoxX[iState] > (430 + 60*iState) AND lrBoxX[iState] <= (461 + 60*iState) THEN
					bBoxPlasticMove[iState] := TRUE;
			END_IF
				// box in wrong position related to the plastic cylinder >> accident
			IF lrBoxX[iState] > (381 + 60*iState) AND lrBoxX[iState] <= (430 + 60*iState)
				AND NOT bStopped THEN
					bAccident := TRUE;
			END_IF	
		END_IF
	END_FOR
END_IF

// =========================================================
END_METHOD

METHOD PRIVATE M_Reset
VAR_INPUT
END_VAR
// =========================================================
	// Resetting visu
	
// Cylinder buttons
bButtonClampToWorkOut := FALSE;
bButtonBarrierToWorkOut := FALSE;
bButtonMetalToWorkOut := FALSE;
bButtonPlasticToWorkOut := FALSE;

// Axis buttons
bButtonMainBwOut := FALSE;
bButtonMainFwOut := FALSE;
bButtonMetalBwOut := FALSE;
bButtonMetalFwOut := FALSE;
bButtonPlasticBwOut := FALSE;
bButtonPlasticFwOut := FALSE;

// State and mode buttons
bButtonStartOut := FALSE;
bButtonStopOut := FALSE;
bButtonResetOut := FALSE;
bButtonComprAirOut := FALSE;
bButtonManuOut := FALSE;
bButtonAutoOut := FALSE;
bButtonSemiOut := FALSE;
bButtonMaintenanceOut := FALSE;

// Position of boxes and cylinders	
FOR iState := 1 TO 4 BY 1 DO
	lrBoxX[iState] := 0;
	lrBoxY[iState] := 0;
	bBoxMetalMove[iState] := FALSE;
	bBoxPlasticMove[iState] := FALSE;
	bBoxMainBelt[iState] := FALSE;
	bBoxMetalBelt[iState] := FALSE;
	bBoxPlasticBelt[iState] := FALSE;
END_FOR

bAccident := FALSE;

// =========================================================
END_METHOD

END_FUNCTION_BLOCK
